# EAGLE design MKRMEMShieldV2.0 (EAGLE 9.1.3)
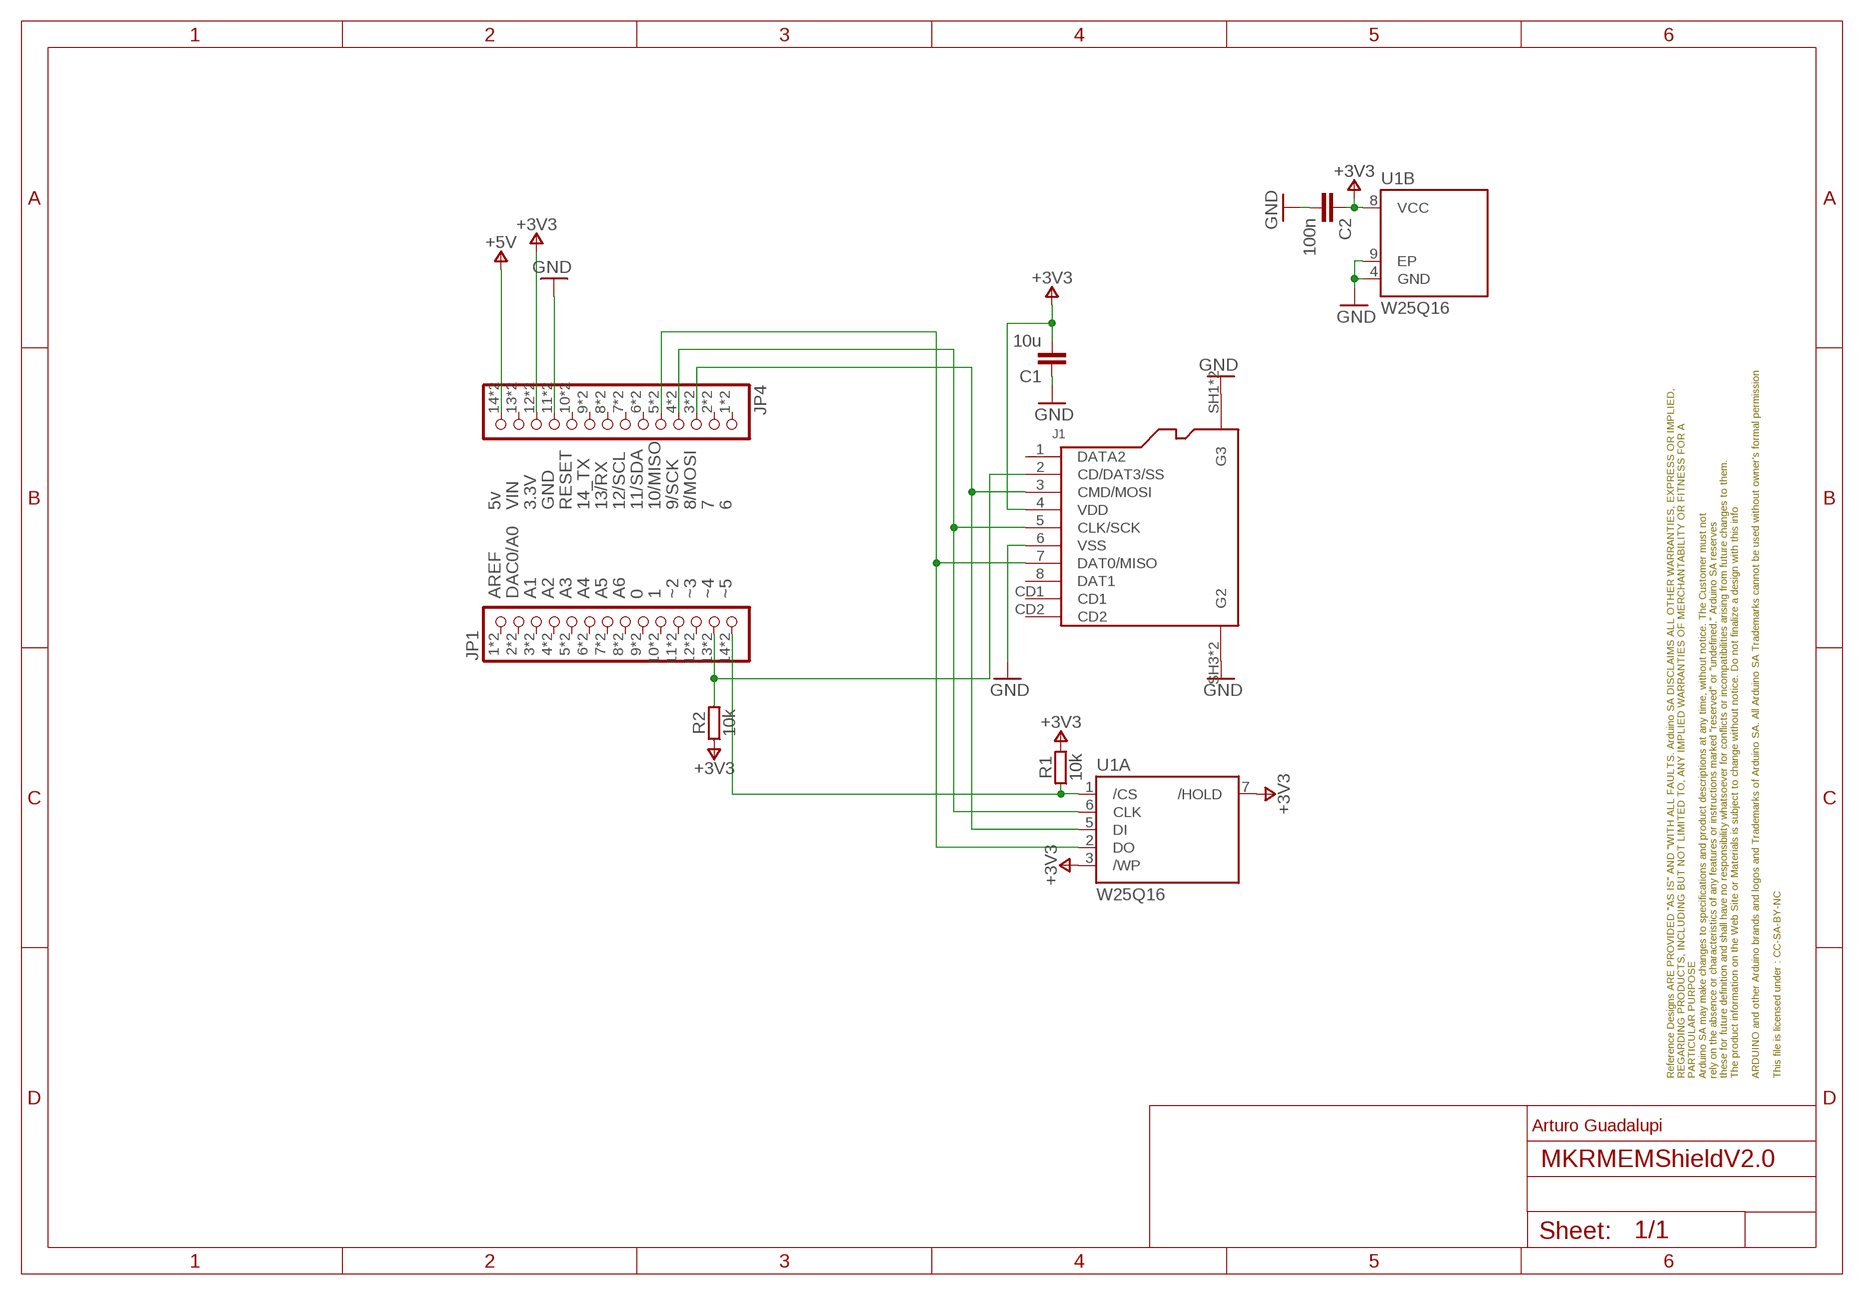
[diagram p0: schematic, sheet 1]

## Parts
C1  10u  C-10UF-0603  [0603-1608X90N]
C2  100n  C-100NF-0603  [0603-1608X90N]
FRAME1  DNP  A4L-LOC  [FRAME]
J1  -  SD_AMPHENOL  [AMPHENOL_114-00841-68]
JP1  -  PINHD-1X14TH-DOUBLE  [1X14-DOUBLE]
JP4  -  PINHD-1X14TH-DOUBLE  [1X14-DOUBLE]
R1  10k  R-10K-0603  [C0603]
R2  10k  R-10K-0603  [C0603]
U1  W25Q16  W25Q16DVZPIG  [SON9P127_500X600X80L60X41T340X400N]

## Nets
+3V3: C1.2 C2.1 J1.4(VDD) JP4.12 JP4.26 R1.2 R2.1 U1.3(A:/WP) U1.7(A:/HOLD) U1.8(B:VCC)
+5V: JP4.14 JP4.28
GND: C1.1 C2.2 J1.6(VSS) J1.SH1(G3) J1.SH2(G3) J1.SH3(G2) J1.SH4(G2) JP4.11 JP4.25 U1.4(B:GND) U1.9(B:EP)
N$1: JP1.14 JP1.28 R1.1 U1.1(A:/CS)
N$3: J1.3(CMD/MOSI) JP4.3 JP4.17 U1.5(A:DI)
N$4: J1.5(CLK/SCK) JP4.4 JP4.18 U1.6(A:CLK)
N$5: J1.7(DAT0/MISO) JP4.5 JP4.19 U1.2(A:DO)
N$77: J1.2(CD/DAT3/SS) JP1.13 JP1.27 R2.2
Unconnected: J1.1(DATA2) J1.8(DAT1) J1.CD1 J1.CD2 JP1.1 JP1.2 JP1.3 JP1.4 JP1.5 JP1.6 JP1.7 JP1.8 JP1.9 JP1.10 JP1.11 JP1.12 JP1.15 JP1.16 JP1.17 JP1.18 JP1.19 JP1.20 JP1.21 JP1.22 JP1.23 JP1.24 JP1.25 JP1.26 JP4.1 JP4.2 JP4.6 JP4.7 JP4.8 JP4.9 JP4.10 JP4.13 JP4.15 JP4.16 JP4.20 JP4.21 JP4.22 JP4.23 JP4.24 JP4.27

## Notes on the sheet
- 5v | VIN | 3.3V | GND | RESET | 14_TX | 13/RX | 12/SCL | 11/SDA | 10/MISO | 9/SCK | 8/MOSI | 7 | 6
- AREF | DAC0/A0 | A1 | A2 | A3 | A4 | A5 | A6 | 0 | 1 | ~2 | ~3 | ~4 | ~5
- Arturo Guadalupi

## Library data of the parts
C1 = Arduino-rcl:C: SMD Capacitor; CODE-BCE: -; CODE-BCMI: -; CODE-TK2: -; DATASHEET: http://www.murata.com/~/media/webrenewal/support/library/catalog/products/capacitor/mlcc/c02e.pdf; DISTRIBUTOR-LINK: http://www.digikey.com/product-search/en?keywords=490-10728-1-ND; DISTRIBUTOR-PN: 490-10728-1-ND; MANUFACTURER: Murata; MANUFACTURER-PN: GRM188R61C106KAALD
C2 = Arduino-rcl:C: SMD Capacitor; CODE-BCE: SP0015; CODE-BCMI: 0015; CODE-TK2: CL10B104KB8NNNC; DATASHEET: http://search.murata.co.jp/Ceramy/image/img/A01X/G101/ENG/GRM188R71C104KA01-01.pdf; DISTRIBUTOR-LINK: https://www.digikey.com/product-detail/en/murata-electronics-north-america/GRM188R71C104KA01D/490-1532-1-ND/587771; DISTRIBUTOR-PN: 490-1532-2-ND; MANUFACTURER: Murata; MANUFACTURER-PN: GRM188R71C104KA01D
FRAME1 = Arduino-utility:A4L-LOC: FRAME; CODE-ARDUINO: DNP; DATASHEET: DNP; DISTRIBUTOR-LINK: DNP; DISTRIBUTOR-PN: DNP; MANUFACTURER: DNP; MANUFACTURER-PN: DNP
J1 = Arduino-connectors:SD_AMPHENOL: Micro SD connector; CODE-BCE: -; CODE-TK2: -; DATASHEET: https://www.amphenolcanada.com/ProductSearch/drawings/AC/1140084168.pdf; DISTRIBUTOR-LINK: http://www.digikey.com/product-detail/en/amphenol-commercial-products/114-00841-68/114-00841-68-1-ND/2187101; DISTRIBUTOR-PN: 114-00841-68-1-ND; MANUFACTURER: Amphenol; MANUFACTURER-PN: 114-00841-68
JP1 JP4 = Arduino-connectors:PINHD-1X14: PIN HEADER; CODE-BCE: -; CODE-TK2: -; DATASHEET: -; DISTRIBUTOR-LINK: -; DISTRIBUTOR-PN: -; MANUFACTURER: ELDECO; MANUFACTURER-PN: FH254114DF08500T
R1 R2 = Arduino-rcl:R: SMD Resistor; CODE-BCE: SP0899; CODE-BCMI: 0899; CODE-TK2: -; DATASHEET: http://www.yageo.com/documents/recent/PYu-RC_Group_51_RoHS_L_8.pdf; DISTRIBUTOR-LINK: https://www.digikey.com/product-detail/en/yageo/RC0603JR-0710KL/311-10KGRCT-ND/729647; DISTRIBUTOR-PN: 311-10KGRCT-ND; MANUFACTURER: Yageo; MANUFACTURER-PN: RC0603JR-0710KL
U1 = Arduino-ICs:W25Q*: Flash; CODE-BCE: -; CODE-TK2: -; DATASHEET: https://www.winbond.com/resource-files/w25q16jv%20spi%20revd%2008122016.pdf; DISTRIBUTOR-LINK: https://www.digikey.com/product-detail/it/winbond-electronics/W25Q16JVZPIQ/W25Q16JVZPIQ-ND/6193770; DISTRIBUTOR-PN: W25Q16JVZPIQ-ND; MANUFACTURER: Winbond; MANUFACTURER-PN: W25Q16JVZPIQ

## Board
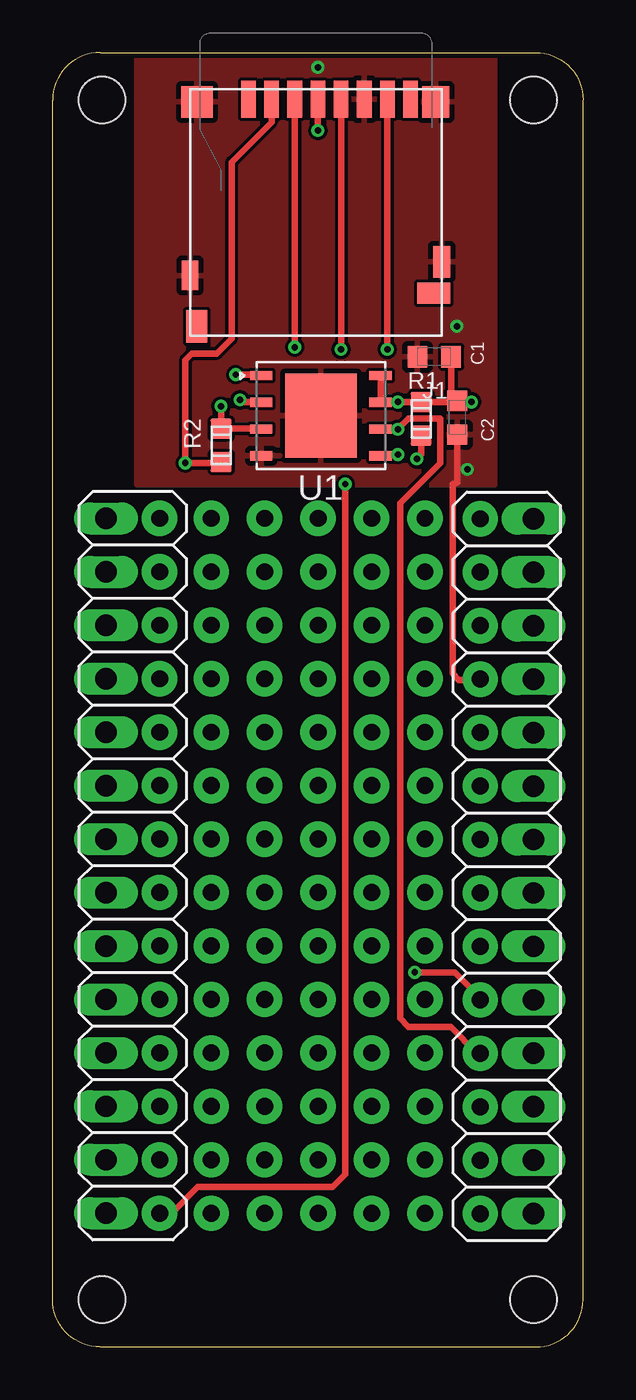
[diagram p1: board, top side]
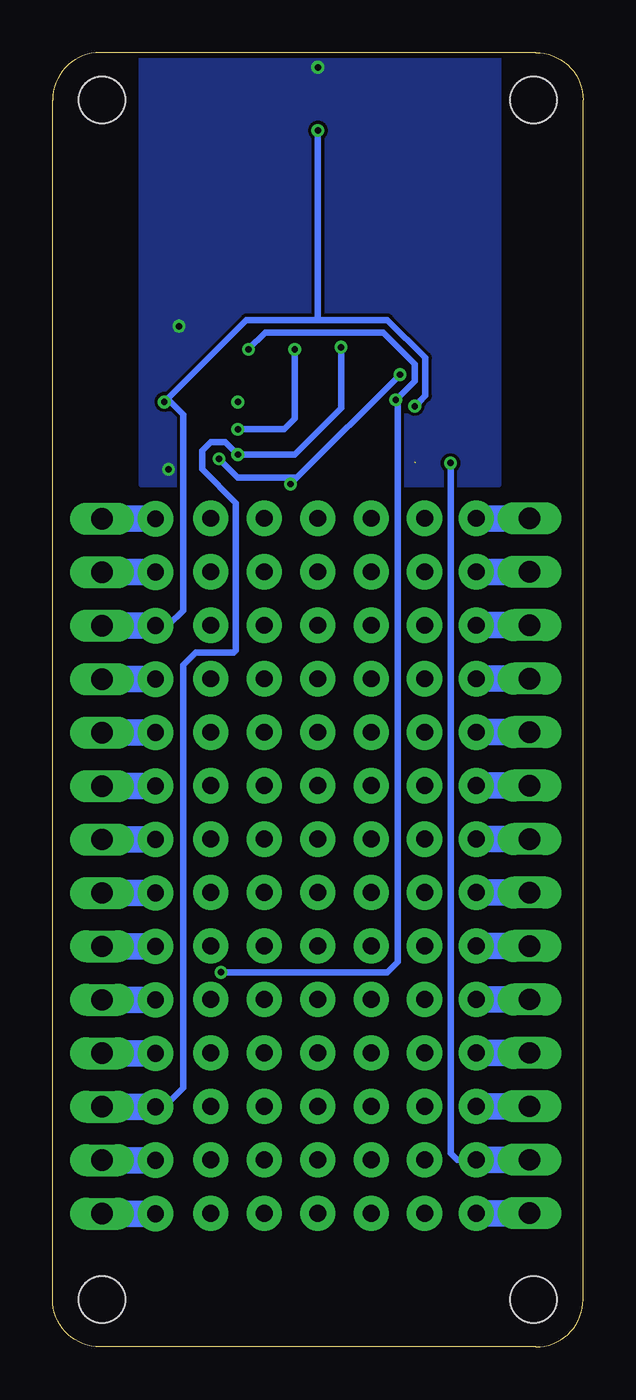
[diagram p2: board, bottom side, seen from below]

Size 25.2 x 61.5 mm. Coordinates in mm from the lower left corner, seen from the top.
Outline: 25.2,2.25 25.2,59.25 arc90 22.95,61.5 2.25,61.5 arc90 0,59.25 0,2.25 arc90 2.25,0 22.95,0 arc90 25.2,2.25
Copper layers (1*16): Top 0.035mm / dielectric 1.5mm / Bottom 0.035mm
Design rules "SeeedStudio_2layers": minimum track width 6mil, minimum drill 12mil, track to track 6mil, track to pad 6mil, pad to pad 6mil, via to via 6mil, smd to smd 0mil, copper to edge 10mil, drill to drill 10mil, minimum pad ring 10mil, minimum via ring 6mil, stop-mask expansion 2mil, vias tented up to drill 100mil, thermal gap 10mil
Holes 2.2 mm at 2.35,2.25 22.85,2.25 2.35,59.25 22.85,59.25

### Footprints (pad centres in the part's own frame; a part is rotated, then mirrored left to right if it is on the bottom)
0603-1608X90N = smd 0.95 x 1: 1 -0.8,0; 2 0.8,0
AMPHENOL_114-00841-68 = smd 0.7 x 1.75: 1 3.2,-5.888; 2 2.1,-5.888; 3 1,-5.888; 4 -0.1,-5.888; 5 -1.2,-5.888; 6 -2.3,-5.888; 7 -3.4,-5.888; 8 -4.5,-5.888 | smd 1 x 1.55: CD1 5.65,4.912 | smd 1.55 x 1: CD2 -5.602,3.337 | smd 1.3 x 1.5: SH1 -5.7,-5.76 | smd 1.5 x 1.5: SH2 5.65,-5.76 | smd 0.8 x 1.4: SH3 5.975,2.487 | smd 0.8 x 1.5: SH4 -5.975,1.837
1X14-DOUBLE = drill 1.016 long: 1 -16.51,0; 2 -13.97,0; 3 -11.43,0; 4 -8.89,0; 5 -6.35,0; 6 -3.81,0; 7 -1.27,0; 8 1.27,0; 9 3.81,0; 10 6.35,0; 11 8.89,0; 12 11.43,0; 13 13.97,0; 14 16.51,0 | drill 0.8 pad 1.676: 15 -16.51,2.54; 16 -13.97,2.54; 17 -11.43,2.54; 18 -8.89,2.54; 19 -6.35,2.54; 20 -3.81,2.54; 21 -1.27,2.54; 22 1.27,2.54; 23 3.81,2.54; 24 6.35,2.54; 25 8.89,2.54; 26 11.43,2.54; 27 13.97,2.54; 28 16.51,2.54
C0603 = smd 1 x 0.95: 1 0,0.8; 2 0,-0.8
SON9P127_500X600X80L60X41T340X400N = smd 0.44 x 1.06: 1 -1.905,-2.835; 2 -0.635,-2.835; 3 0.635,-2.835; 4 1.905,-2.835; 5 1.905,2.835; 6 0.635,2.835; 7 -0.635,2.835; 8 -1.905,2.835 | smd 4 x 3.4: 9 0,0

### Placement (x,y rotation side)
C1  18.13,47.05 0 top
C2  19.22,44.15 270 top
FRAME1  not placed on the board
J1  12.5,53.4 180 top
JP1  2.54,22.86 270 top
JP4  22.85,22.84 90 top
R1  17.5,44.1 180 top
R2  8,42.84 0 top
U1  12.74,44.25 270 top

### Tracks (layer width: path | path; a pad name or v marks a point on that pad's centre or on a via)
+3V3  (via drill 0.3)
  Top 0.305: U1.3 9.88,43.64 R2.1 v8,44.7 | U1.8 U1.7 16.39,44.88 v16.4,44.9 R1.2 18.87,44.9 | 18.87,44.9 C2.1 18.93,44.96 C1.2 | 18.87,44.9 v19.9,44.9 | J1.4 v12.6,57.8
  Bottom 0.305: 7.7,45 v8,44.7 7.5,45.2 7.5,47 9.3,48.8 12.6,48.8 | JP4.26 20.28,34.3 19.7,34.3 19,35 19,44.3 19.6,44.9 v19.9,44.9 16,48.8 12.6,48.8 | v12.6,57.8 12.6,48.8
GND  (via drill 0.3)
  Top 0.305: C2.2 19.22,41.08 19,41 19,32 19.3,31.7 20.28,31.7 JP4.25
  other vias: 12.6,60.8 19.7,41.7 19.2,48.5
  pour Top: 21,62.3 21,40.98 4,40.98 4,62.3
  pour Bottom: 21,62.3 21,40.98 4,40.98 4,62.3
N$1  (via drill 0.3)
  Top 0.305: v8.7,46.2 9.86,46.2 U1.1 | R1.1 17.5,42.4 v17.3,42.2 | v13.9,41 13.9,8.2 13.3,7.6 6.9,7.6 5.65,6.35 JP1.28
  Bottom 0.305: 13.6,41.3 v8.7,46.2 | 13.6,41.3 16.4,41.3 v17.3,42.2 | 13.6,41.3 v13.9,41
N$3  (via drill 0.3)
  Top 0.305: J1.3 v11.5,47.5 | U1.5 16.34,42.34 v16.4,42.4
  Bottom 0.305: v11.5,47.5 11.5,44.6 13.7,42.4 v16.4,42.4 17,43 17.7,43 18.1,42.6 18.1,41.7 16.5,40.1 16.5,33.1 16.6,33 18.4,33 19,32.4 19,12.3 19.89,11.41 JP4.17
N$4  (via drill 0.3)
  Top 0.305: J1.5 v13.7,47.4 | U1.6 16.39,43.62 v16.4,43.6 16.9,44.1 18.4,44.1 18.4,42 16.5,40.1 16.5,15.6 16.9,15.2 18.9,15.2 20.15,13.95 JP4.18
  Bottom 0.305: v16.4,43.6 14.2,43.6 13.7,44.1 v13.7,47.4
N$5  (via drill 0.3)
  Top 0.305: J1.7 v15.9,47.4 | U1.2 9.02,44.88 v8.9,45 | JP4.19 20.31,16.59 19.1,17.8 v17.2,17.8
  Bottom 0.305: v15.9,47.4 15.1,48.2 9.5,48.2 8,46.7 8,45.9 v8.9,45 8.8,44.9 8.8,18.3 9.3,17.8 v17.2,17.8
N$6  (via drill 0.8 pad 1.68)
  other vias: 7.53,31.75
N$7  (via drill 0.8 pad 1.68)
  other vias: 7.53,34.29
N$8  (via drill 0.8 pad 1.68)
  other vias: 10.07,34.29
N$9  (via drill 0.8 pad 1.68)
  other vias: 10.07,29.21
N$10  (via drill 0.8 pad 1.68)
  other vias: 17.69,6.35
N$11  (via drill 0.8 pad 1.68)
  other vias: 12.61,29.21
N$12  (via drill 0.8 pad 1.68)
  other vias: 17.69,29.21
N$13  (via drill 0.8 pad 1.68)
  other vias: 7.53,36.83
N$14  (via drill 0.8 pad 1.68)
  other vias: 17.69,36.83
N$15  (via drill 0.8 pad 1.68)
  other vias: 10.07,31.75
N$16  (via drill 0.8 pad 1.68)
  other vias: 12.61,31.75
N$17  (via drill 0.8 pad 1.68)
  other vias: 17.69,31.75
N$18  (via drill 0.8 pad 1.68)
  other vias: 17.69,26.67
N$19  (via drill 0.8 pad 1.68)
  other vias: 12.61,26.67
N$20  (via drill 0.8 pad 1.68)
  other vias: 10.07,26.67
N$21  (via drill 0.8 pad 1.68)
  other vias: 7.53,29.21
N$22  (via drill 0.8 pad 1.68)
  other vias: 7.53,19.05
N$23  (via drill 0.8 pad 1.68)
  other vias: 10.07,36.83
N$24  (via drill 0.8 pad 1.68)
  other vias: 7.53,39.37
N$25  (via drill 0.8 pad 1.68)
  other vias: 10.07,39.37
N$26  (via drill 0.8 pad 1.68)
  other vias: 15.15,6.35
N$27  (via drill 0.8 pad 1.68)
  other vias: 15.15,8.89
N$28  (via drill 0.8 pad 1.68)
  other vias: 15.15,11.43
N$29  (via drill 0.8 pad 1.68)
  other vias: 15.15,13.97
N$30  (via drill 0.8 pad 1.68)
  other vias: 15.15,19.05
N$31  (via drill 0.8 pad 1.68)
  other vias: 15.15,21.59
N$32  (via drill 0.8 pad 1.68)
  other vias: 15.15,16.51
N$33  (via drill 0.8 pad 1.68)
  other vias: 15.15,24.13
N$34  (via drill 0.8 pad 1.68)
  other vias: 10.07,21.59
N$35  (via drill 0.8 pad 1.68)
  other vias: 12.61,21.59
N$36  (via drill 0.8 pad 1.68)
  other vias: 17.69,24.13
N$37  (via drill 0.8 pad 1.68)
  other vias: 12.61,24.13
N$38  (via drill 0.8 pad 1.68)
  other vias: 10.07,24.13
N$39  (via drill 0.8 pad 1.68)
  other vias: 7.53,26.67
N$40  (via drill 0.8 pad 1.68)
  other vias: 7.53,21.59
N$41  (via drill 0.8 pad 1.68)
  other vias: 7.53,24.13
N$42  (via drill 0.8 pad 1.68)
  other vias: 10.07,19.05
N$43  (via drill 0.8 pad 1.68)
  other vias: 12.61,19.05
N$44  (via drill 0.8 pad 1.68)
  other vias: 17.69,21.59
N$45  (via drill 0.8 pad 1.68)
  other vias: 17.69,19.05
N$46  (via drill 0.8 pad 1.68)
  other vias: 12.61,16.51
N$47  (via drill 0.8 pad 1.68)
  other vias: 10.07,16.51
N$48  (via drill 0.8 pad 1.68)
  other vias: 10.07,13.97
N$49  (via drill 0.8 pad 1.68)
  other vias: 12.61,13.97
N$51  (via drill 0.8 pad 1.68)
  other vias: 12.61,11.43
N$52  (via drill 0.8 pad 1.68)
  other vias: 10.07,11.43
N$53  (via drill 0.8 pad 1.68)
  other vias: 10.07,8.89
N$54  (via drill 0.8 pad 1.68)
  other vias: 12.61,8.89
N$55  (via drill 0.8 pad 1.68)
  other vias: 17.69,16.51
N$56  (via drill 0.8 pad 1.68)
  other vias: 17.69,13.97
N$57  (via drill 0.8 pad 1.68)
  other vias: 17.69,11.43
N$58  (via drill 0.8 pad 1.68)
  other vias: 17.69,8.89
N$59  (via drill 0.8 pad 1.68)
  other vias: 12.61,6.35
N$60  (via drill 0.8 pad 1.68)
  other vias: 10.07,6.35
N$61  (via drill 0.8 pad 1.68)
  other vias: 15.15,26.67
N$62  (via drill 0.8 pad 1.68)
  other vias: 7.53,8.89
N$63  (via drill 0.8 pad 1.68)
  other vias: 7.53,11.43
N$64  (via drill 0.8 pad 1.68)
  other vias: 7.53,13.97
N$65  (via drill 0.8 pad 1.68)
  other vias: 7.53,16.51
N$66  (via drill 0.8 pad 1.68)
  other vias: 7.53,6.35
N$67  (via drill 0.8 pad 1.68)
  other vias: 15.15,29.21
N$68  (via drill 0.8 pad 1.68)
  other vias: 15.15,31.75
N$69  (via drill 0.8 pad 1.68)
  other vias: 15.15,34.29
N$70  (via drill 0.8 pad 1.68)
  other vias: 12.61,34.29
N$71  (via drill 0.8 pad 1.68)
  other vias: 15.15,36.83
N$72  (via drill 0.8 pad 1.68)
  other vias: 12.61,36.83
N$73  (via drill 0.8 pad 1.68)
  other vias: 12.61,39.37
N$74  (via drill 0.8 pad 1.68)
  other vias: 15.15,39.37
N$75  (via drill 0.8 pad 1.68)
  other vias: 17.69,39.37
N$76  (via drill 0.8 pad 1.68)
  other vias: 17.69,34.29
N$77  (via drill 0.3)  (1 unrouted)
  Top 0.305: 7.96,42 v6.3,42 6.3,46.9 6.6,47.2 7.8,47.2 8.5,47.9 8.5,56.3 10.4,58.2 J1.2
  Bottom 0.305: v6.3,42 6.3,9.2 5.99,8.89 JP1.27

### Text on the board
Notes: Arturo Guadalupi

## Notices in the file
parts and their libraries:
Arduino-ICs: Copyright (c) 2016-2017 Arduino LLC. All right reserved.
Arduino-utility: This file is licensed under : CC-SA-BY-NC
